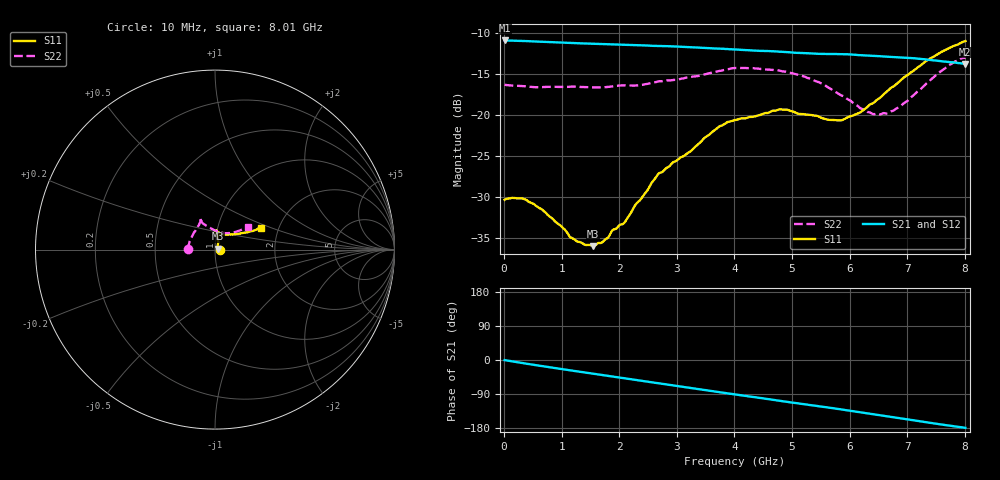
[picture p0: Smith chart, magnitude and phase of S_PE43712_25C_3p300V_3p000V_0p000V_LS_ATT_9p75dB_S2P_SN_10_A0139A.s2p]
! DEVICE ID: PE43712
! File Path: z:\PE43713\PE43713_CHAR_NOM_04292014\AMB\3p300\LS_ATT_9p75dB\PE43713_AMB_3p300V_3p000V_0p000V_LS_ATT_9p75dB_S2P_SN_10_A0139A.s2p
! Serial: 10
! Lot: A0139A
! Temp: 25C
! VDD: 3.300
! VSS: 0.000
! Control_Hi: 3.000
! Control_Lo: 0.000
! Attenuation Step: 9.75dB
! Port 1: RF1
! Port 2: RF2
! ThroughPath:1-2
! IDD: 0.0001469322
! ISS: -7.72e-008
#  Hz  S  RI  R  50
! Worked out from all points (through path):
!   801 points, 10 MHz to 8.01 GHz, reference 50 ohm
!   highest |S21| = -10.92 dB at 10 MHz (marker M1); lowest = -13.8 dB at 8 GHz (marker M2)
!   group delay of S21, straight-line fit = 61.5 ps
!   lowest |S11| = -36.0 dB at 1.54 GHz (marker M3), VSWR 1.03, Z = 51.5 + j0.505 ohm
!   |S11| at or under -10 dB: start of sweep to end of sweep
!   |S22| runs from -19.9 to -13.0 dB; largest |S21 - S12| = 0.001
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1e7  0.0304 0.000124  0.2845 -0.00158  0.2847 -0.00145  -0.1528 0.000981
3e8  0.0308 -0.00356  0.2801 -0.0372  0.2801 -0.0372  -0.1491 0.0149
5e8  0.0284 -0.00475  0.2743 -0.0603  0.2744 -0.0602  -0.1463 0.0233
1.01e9  0.0205 -0.00246  0.2516 -0.1131  0.2518 -0.1131  -0.1408 0.0464
1.17e9  0.0178 -0.000631  0.2428 -0.1276  0.2428 -0.1278  -0.1386 0.0537
1.35e9  0.0165 0.00147  0.2322 -0.1436  0.2322 -0.1437  -0.135 0.0606
1.54e9  0.0151 0.0049  0.2199 -0.1595  0.2199 -0.1596  -0.1295 0.0697
1.72e9  0.0144 0.00883  0.2074 -0.1737  0.2074 -0.1737  -0.1252 0.0776
2.09e9  0.0135 0.0174  0.1787 -0.1998  0.1787 -0.1997  -0.1179 0.0948
2.68e9  0.0185 0.0397  0.1265 -0.2308  0.1264 -0.2308  -0.0959 0.1284
3.72e9  0.0128 0.0831  0.0246 -0.2525  0.0245 -0.2524  -0.0813 0.1658
4.01e9  0.00963 0.0926  -0.00363 -0.2508  -0.00366 -0.2508  -0.0841 0.1739
4.79e9  0.00508 0.1082  -0.0738 -0.2314  -0.0738 -0.2317  -0.0804 0.1678
5.35e9  0.0159 0.0982  -0.1169 -0.2062  -0.1169 -0.2061  -0.0704 0.1488
5.88e9  0.039 0.0848  -0.1541 -0.1769  -0.1538 -0.1769  -0.0354 0.1258
6.39e9  0.081 0.0847  -0.1819 -0.1396  -0.1815 -0.1395  0.0137 0.1009
6.68e9  0.1134 0.0861  -0.1941 -0.1161  -0.1938 -0.1162  0.0466 0.0921
6.99e9  0.1474 0.0916  -0.2043 -0.0898  -0.2039 -0.0897  0.0786 0.0917
7.35e9  0.1906 0.1002  -0.2096 -0.0572  -0.2094 -0.0572  0.1204 0.1012
7.72e9  0.2297 0.111  -0.2087 -0.0257  -0.2086 -0.0258  0.1627 0.1169
8e9  0.2532 0.1219  -0.2046 -0.00454  -0.2044 -0.00486  0.1835 0.127
8.01e9  0.254 0.1226  -0.2046 -0.00399  -0.2043 -0.00433  0.1841 0.1273
